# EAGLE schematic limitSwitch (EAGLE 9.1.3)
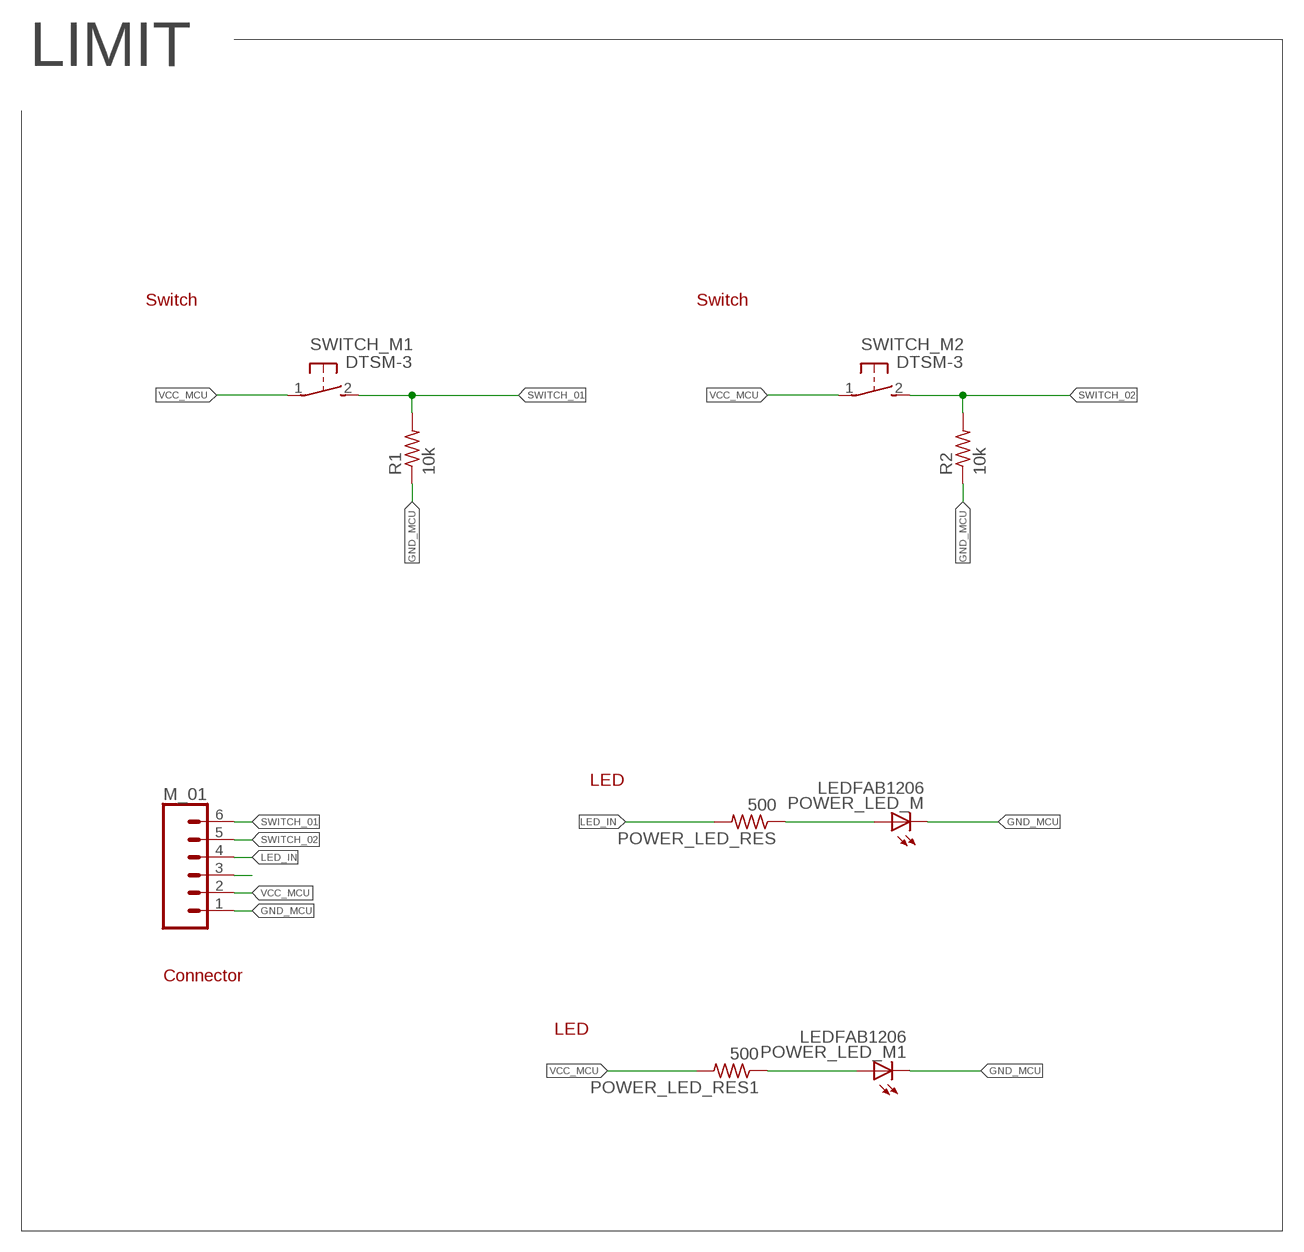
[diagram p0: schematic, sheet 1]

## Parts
M_01  CONN_06SMD-1MM  [1X06-1MM]
POWER_LED_M  LEDFAB1206  [LED1206FAB]
POWER_LED_M1  LEDFAB1206  [LED1206FAB]
POWER_LED_RES  500  R-US_M0805  [M0805]
POWER_LED_RES1  500  R-US_M0805  [M0805]
R1  10k  R-US_M0805  [M0805]
R2  10k  R-US_M0805  [M0805]
SWITCH_M1  DTSM-3  [DTSM-3]
SWITCH_M2  DTSM-3  [DTSM-3]

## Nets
GND_MCU: M_01.1 POWER_LED_M1.2(C) POWER_LED_M.2(C) R1.1 R2.1
LED_IN: M_01.4 POWER_LED_RES.2
N$1: POWER_LED_M1.1(A) POWER_LED_RES1.1
N$11: POWER_LED_M.1(A) POWER_LED_RES.1
NEO_PIXEL: M_01.3
SWITCH_01: M_01.6 R1.2 SWITCH_M1.2
SWITCH_02: M_01.5 R2.2 SWITCH_M2.2
VCC_MCU: M_01.2 POWER_LED_RES1.2 SWITCH_M1.1 SWITCH_M2.1

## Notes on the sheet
- LIMIT
- Switch | Switch
- LED
- Connector
- LED

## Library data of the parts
M_01 = SparkFun-Connectors:CONN_06: Multi connection point. Often used as Generic Header-pin footprint for 0.1 inch spaced/style header connections On any of the 0.1 inch spaced packages, you can populate with these: Break Away Headers - Straight (PRT-00116) Break Away Male Headers - Right Angle (PRT-00553) Female Headers (PRT-00115)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; PROD_ID: CONN-08249; SF_ID: GPS-00579
POWER_LED_M POWER_LED_M1 = fab:LED: LED
POWER_LED_RES POWER_LED_RES1 R1 R2 = resistor:R-US_: RESISTOR, American symbol
SWITCH_M1 SWITCH_M2 = switch-tact:DTSM-3

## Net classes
0 default: width 0.2 mm, clearance 0.12 mm

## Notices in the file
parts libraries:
SparkFun-Connectors: Licensing: Creative Commons ShareAlike 4.0 International - https://creativecommons.org/licenses/by-sa/4.0
